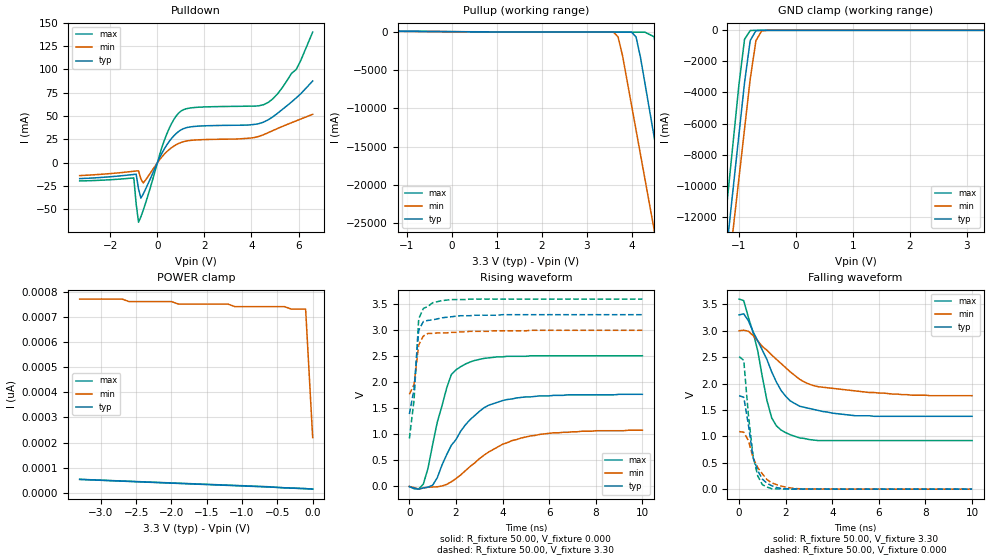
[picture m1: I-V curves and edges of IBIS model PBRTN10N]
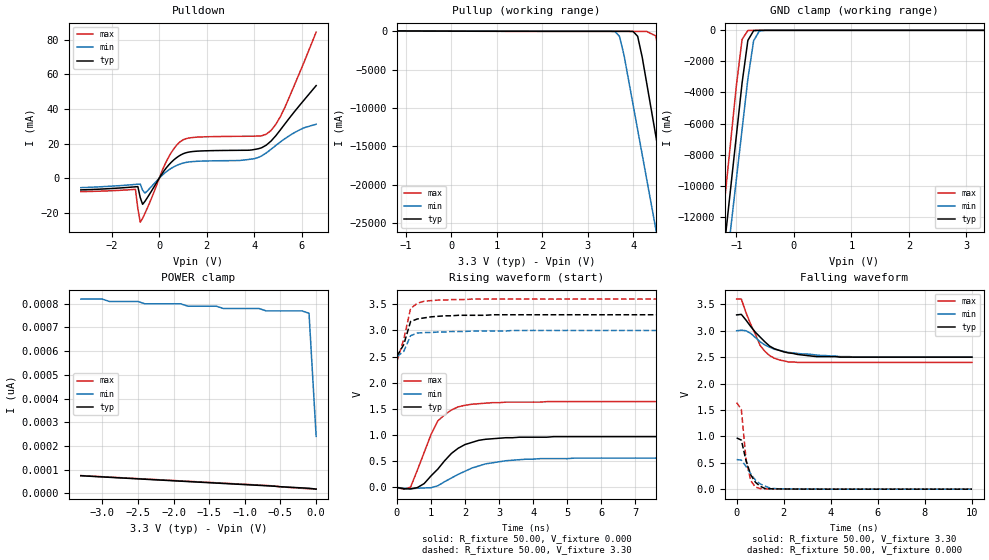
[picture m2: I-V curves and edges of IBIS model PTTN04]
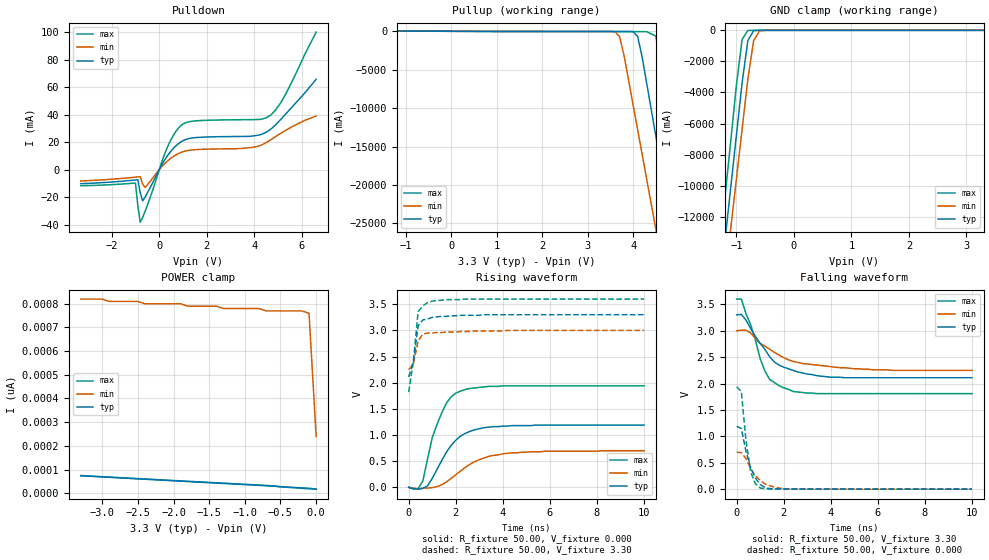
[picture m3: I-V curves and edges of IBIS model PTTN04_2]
| Integrated Devices Technolgy, Inc.
| IBIS MODEL OF 82v2048E
| BGA_208
[Ibis Ver]   2.1
[File Name]   2048E_02.ibs
[File Rev]   1.0
[Date]   10/24/2002
[Source]   Integrated Devices Technolgy, Inc.
[Notes]   Spice type : spectre
[Disclaimer] Integrated Device Technology, Inc. ("IDT") hereby grants the
   user of this IBIS model a non-exclusive, nontransferable
   license to use this IBIS model under the following terms. The
   user is granted this license only to use the IBIS model and is
   not granted rights to sell, copy (except as needed to run the
   IBIS model), rent, lease or sub-license the IBIS model in
   whole or in part, or in modified form to anyone. The User may
   modify the IBIS model to suit its specific applications, but
   rights to derivative works and such modifications shall belong
   to IDT. This IBIS model is provided on an AS IS" basis and IDT
   makes absolutely no warranty with respect to the information
   contained herein. IDT DISCLAIMS AND CUSTOMER WAIVES ALL
   WARRANTIES, EXPRESS AND IMPLIED, INCLUDING WARRANTIES OF
   MERCHANTABILITY AND FITNESS FOR A PARTICULAR PURPOSE. THE
   ENTIRE RISK AS TO QUALITY AND PERFORMANCE IS WITH THE USER
   ACCORDINGLY, IN NO EVENT SHALL IDT BE LIABLE FOR ANY DIRECT OR
   INDIRECT DAMAGES, WHETHER IN CONTRACT OR TORT, INCLUDING ANY
   LOST PROFITS OR OTHER INCIDENTAL, CONSEQUENTIAL, EXEMPLARY, OR
   PUNITIVE DAMAGES ARISING OUT OF THE USE OR APPLICATION OF THE
   IBIS model. Further, IDT reserves the right to make changes
   without notice to any product herein to improve reliability,
   function, or design. IDT does not convey any license under
   patent rights or any other intellectual property rights,
   including those of third parties. IDT is not obligated to
   provide maintenance or support for the licensed IBIS model.
[Copyright]   Copyright 2002, Integrated Devices Technolgy, Inc. all rights
   reserved
|   Component 2048E_02 (BGA_208)
[Component]   2048E_02
[Manufacturer]   Integrated Devices Technolgy, Inc.
[Package]
| variable   typ   min   max
R_pkg   169.8m   150.2m   189.4m
L_pkg   4.44nH   3.68nH   5.19nH
C_pkg   0.81pF   0.54pF   1.08pF
|   Pin List ( BGA_208 )
[PIN]   signal_name   Model_name   R_pin   L_pin   C_pin
   A1   GNDA   GND
   A2   GNDT4   GND
   A3   TTIP4   DRIVER
   A4   VDDT   POWER
   A5   RTIP4   PAI
   A6   TRST   PITSU
   A7   GNDT2   GND
   A8   TTIP2   DRIVER
   A9   VDDT   POWER
   A10   TCK   PITSN
   A11   RTIP2   PAI
   A12   GNDT1   GND
   A13   TTIP1   DRIVER
   A14   VDDT   POWER
   A15   TCLK1   PITSN
   A16   RCLK1   PTTN04_2
   B1   SCLKE   PITSN
   B2   GNDT12   GND
   B3   TRING4   DRIVER
   B4   VDDT   POWER
   B5   RRING4   PAI
   B6   TMS   PITSU
   B7   GNDT10   GND
   B8   TRING2   DRIVER
   B9   VDDT   POWER
   B10   TDO   PTTN04
   B11   RRING2   PAI
   B12   GNDT9   GND
   B13   TRING1   DRIVER
   B14   VDDT   POWER
   B15   TD1/TDP1   PITSN
   B16   RD1/RDP1   PTTN04
   C1   VDDA   POWER
   C2   LOS1   POTN04
   C3   LOS2   POTN04
   C4   VDDR4   POWER
   C5   RTIP3   PAI
   C6   GNDR4   GND
   C7   GNDT3   GND
   C8   TTIP3   DRIVER
   C9   VDDT   POWER
   C10   VDDR2   POWER
   C11   RTIP1   PAI
   C12   GNDR2   GND
   C13   NC   NC
   C14   TDN1   PITSN
   C15   CV1/RDN1   PTTN04
   C16   TCLK2   PITSN
   D1   LOS3   POTN04
   D2   LOS4   POTN04
   D3   LOS5   POTN04
   D4   VDDR3   POWER
   D5   RRING3   PAI
   D6   GNDR3   GND
   D7   GNDT11   GND
   D8   TRING3   DRIVER
   D9   VDDT   POWER
   D10   VDDR1   POWER
   D11   RRING1   PAI
   D12   GNDR1   GND
   D13   TDI   PITSU
   D14   TDN2   PITSN
   D15   TD2/TDP2   PITSN
   D16   RCLK2   PTTN04_2
   E1   LOS6   POTN04
   E2   LOS7   POTN04
   E3   LOS8   POTN04
   E4   THZ   PITSN
   E13   CV2/RDN2   PTTN04
   E14   RD2/RDP2   PTTN04
   E15   TD3/TDP3   PITSN
   E16   TCLK3   PITSN
   F1   VDDD   POWER
   F2   INT/MOT   PITSN
   F3   IC   PITSN
   F4   GNDD   GND
   F13   TDN3   PITSN
   F14   CV3/RDN3   PTTN04
   F15   RD3/RDP3   PTTN04
   F16   RCLK3   PTTN04_2
   G1   MCLK   PITSN
   G2   GPIO0   PBRTN10N
   G3   GPIO1   PBRTN10N
   G4   P/S   PITSN
   G7   GNDA   GND
   G8   NC   NC
   G9   VDDIO   POWER
   G10   VDDIO   POWER
   G13   GNDD   GND
   G14   TDN4   PITSN
   G15   TD4/TDP4   PITSN
   G16   TCLK4   PITSN
   H1   VDDIO   POWER
   H2   D6   PBRTN10N
   H3   D7   PBRTN10N
   H4   GNDIO   GND
   H7   GNDA   GND
   H8   GNDA   GND
   H9   NC   NC
   H10   NC   NC
   H13   CV4/RDN4   PTTN04
   H14   RD4/RDP4   PTTN04
   H15   RCLK4   PTTN04_2
   H16   VDDD   POWER
   J1   D5   PBRTN10N
   J2   D4   PBRTN10N
   J3   D3   PBRTN10N
   J4   D2   PBRTN10N
   J7   GNDA   GND
   J8   GNDA   GND
   J9   GNDIO   GND
   J10   GNDIO   GND
   J13   GNDIO   GND
   J14   TDN5   PITSN
   J15   TD5/TDP5   PITSN
   J16   TCLK5   PITSN
   K1   VDDIO   POWER
   K2   D0   PBRTN10N
   K3   D1   PBRTN10N
   K4   GNDIO   GND
   K7   GNDA   GND
   K8   GNDA   GND
   K9   GNDA   GND
   K10   GNDA   GND
   K13   CV5/RDN5   PTTN04
   K14   RD5/RDP5   PTTN04
   K15   RCLK5   PTTN04_2
   K20   VDDIO   POWER
   L1   A7   PITSN
   L2   A6   PITSN
   L3   A5   PITSN
   L4   A4   PITSN
   L13   TESTV   PAO
   L14   TDN6   PITSN
   L15   TD6/TDP6   PITSN
   L16   TCLK6   PITSN
   M1   A0   PITSN
   M2   A1   PITSN
   M3   A2   PITSN
   M4   A3   PITSN
   M13   TDN7   PITSN
   M14   CV6/RDN6   PTTN04
   M15   RD6/RDP6   PTTN04
   M16   RCLK6   PTTN04_2
   N1   CS   PITSN
   N2   SCLK   PITSN
   N3   DS/RD   PITSN
   N4   VDDR6   POWER
   N5   RRING6   PAI
   N6   GNDR6   GND
   N7   GNDT6   GND
   N8   TRING6   DRIVER
   N9   VDDT   POWER
   N10   VDDR8   POWER
   N11   RRING8   PAI
   N12   GNDR8   GND
   N13   CV7/RDN7   PTTN04
   N14   RD7/RDP7   PTTN04
   N15   TD7/TDP7   PITSN
   N16   TCLK7   PITSN
   P1   SDI/RW/WR   PITSN
   P2   SDO   PTTN04_2
   P3   RST   PITSU
   P4   VDDR5   POWER
   P5   RTIP6   PAI
   P6   GNDR5   GND
   P7   GNDT14   GND
   P8   TTIP6   DRIVER
   P9   VDDT   POWER
   P10   VDDR7   POWER
   P11   RTIP8   PAI
   P12   GNDR7   GND
   P13   TESTSE   PITSN
   P14   RD8/RDP8   PTTN04
   P15   TDN8   PITSN
   P16   RCLK7   PTTN04_2
   R1   INT   POTN04
   R2   GNDT5   GND
   R3   TRING5   DRIVER
   R4   VDDT   POWER
   R5   RRING5   PAI
   R6   MCLKS   PITSN
   R7   GNDT7   GND
   R8   TRING7   DRIVER
   R9   VDDT   POWER
   R10   TESTAPLL   POTN04
   R11   RRING7   PAI
   R12   GNDT8   GND
   R13   TRING8   DRIVER
   R14   VDDT   POWER
   R15   CV8/RDN8   PTTN04
   R16   TD8/TDP8   PITSN
   T1   REF   PAO
   T2   GNDT13   GND
   T3   TTIP5   DRIVER
   T4   VDDT   POWER
   T5   RTIP5   PAI
   T6   GNDA   GND
   T7   GNDT15   GND
   T8   TTIP7   DRIVER
   T9   VDDT   POWER
   T10   VDDA   POWER
   T11   RTIP7   PAI
   T12   GNDT16   GND
   T13   TTIP8   DRIVER
   T14   VDDT   POWER
   T15   RCLK8   PTTN04_2
   T16   TCLK8   PITSN
| Models and submodels in the file (9): PBRTN10N (I/O), PTTN04 (3-state), PTTN04_2 (3-state), POTN04 (Output), PITSN (Input), PAI (Input), PITSU (Input), PAO (Input), DRIVER (3-state)
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|   Model PBRTN10N
[Model]   PBRTN10N
Model_type   I/O
Polarity   Non-Inverting
Enable   Active-Low
Vinl =   0.74V
Vinh =   2.10V
C_comp   3.50pF   4.00pF   3.20pF
[Temperature Range]   25.00   85.00   -40.00
[Voltage Range]   3.30V   3.00V   3.60V
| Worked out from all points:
|   slope of the pulldown table from 0 to 0.495 V, typ, clamps not added: 21.9 ohm
|   slope of the pullup table from 0 to 0.495 V, typ, clamps not added: 29.2 ohm
|   GND clamp passes 1 mA (typ) near -0.60 V on its own axis
|   rising waveform, R_fixture 50.00, V_fixture 0.000: 20-80 % time 1.59ns typ, 2.13ns min, 825ps max; typ from -0.002 V to 1.77 V
|   rising waveform, R_fixture 50.00, V_fixture 3.30: 20-80 % time 226ps typ, 225ps min, 235ps max; typ from 1.39 V to 3.3 V
|   falling waveform, R_fixture 50.00, V_fixture 3.30: 20-80 % time 1.32ns typ, 1.97ns min, 801ps max; typ from 3.3 V to 1.38 V
|   falling waveform, R_fixture 50.00, V_fixture 0.000: 20-80 % time 472ps typ, 702ps min, 384ps max; typ from 1.77 V to 0 V
[Pulldown]
| voltage   I(typ)   I(min)   I(max)
-3.3V     -16.95mA   -13.71mA   -19.45mA
-1V       -12.5mA    -9.06mA    -16.2mA
-900mV    -12.2mA    -8.75mA    -44.01mA
-800mV    -27.97mA   -8.57mA    -63.62mA
-700mV    -37.8mA    -17.39mA   -57.93mA
-600mV    -33.43mA   -21.55mA   -50.78mA
300mV     15.03mA    9.35mA     24.27mA
900mV     33.46mA    20.65mA    53.15mA
1.5V      38.77mA    24.19mA    59.03mA
4.7V      45.89mA    32.14mA    64.49mA
5.9V      69.46mA    44.93mA    100mA
6.6V      87.62mA    51.95mA    140mA
[Pullup]
| voltage   I(typ)   I(min)   I(max)
-3.3V     120mA      79.67mA    180mA
3.6V      -41.5mA    -64.51mA   -72.86mA
3.7V      -41.65mA   -690mA     -73.1mA
3.8V      -41.8mA    -3.15A     -73.33mA
4.1V      -690mA     -12.84A    -73.96mA
4.3V      -6.82A     -19.3A     -75.1mA
4.5V      -13.65A    -25.76A    -660mA
4.7V      -20.47A    -32.21A    -7.27A
4.9V      -27.29A    -38.67A    -14.54A
5.1V      -34.12A    -45.13A    -21.81A
5.3V      -40.94A    -51.59A    -29.07A
6.6V      -85.3A     -93.57A    -76.32A
[GND_clamp]
| voltage   I(typ)   I(min)   I(max)
-3.3V     -85.25A    -83.86A    -87.14A
-1.3V     -17.02A    -19.27A    -14.46A
-1.2V     -13.61A    -16.05A    -10.83A
-1.1V     -10.19A    -12.82A    -7.2A
-1V       -6.78A     -9.59A     -3.56A
-900mV    -3.37A     -6.36A     -580mA
-800mV    -650mA     -3.13A     -10.84mA
-700mV    -23.03mA   -670mA     -750uA
-600mV    -570uA     -40.72mA   -46.43uA
-400mV    -420nA     -76.92uA   -33.22nA
3.3V      15.23pA    730pA      12.85pA
[POWER_clamp]
| voltage   I(typ)   I(min)   I(max)
-3.3V     53.95pA    770pA      54.34pA
-2.7V     47.02pA    770pA      47.72pA
-2.6V     45.88pA    760pA      46.62pA
-2V       39.11pA    760pA      40.01pA
-1.9V     37.99pA    750pA      38.91pA
-1.2V     30.19pA    750pA      31.21pA
-1.1V     29.08pA    740pA      30.11pA
-400mV    20.85pA    740pA      20.54pA
-300mV    19.76pA    730pA      19.3pA
-100mV    17.59pA    730pA      17.04pA
0V        15.23pA    220pA      15.99pA
[Ramp]
| variable   typ   min   max
dV/dt_r   1.06/1.42n   0.65/2.13n   1.51/0.80n
dV/dt_f   1.15/1.32n   0.74/1.94n   1.61/0.81n
R_load = 50.00
[Rising Waveform]
R_fixture = 50.00
V_fixture = 0.000
V_fixture_min = 0.000
V_fixture_max = 0.000
| time   V(typ)   V(min)   V(max)
0s        -2.35mV    -1.01mV    -3.76mV
600ps     -28.68mV   -31.05mV   45.89mV
1ns       23.7mV     -11.09mV   810mV
1.6ns     610mV      39.29mV    1.89V
1.8ns     790mV      88.39mV    2.15V
2.2ns     1.06V      220mV      2.3V
3.2ns     1.51V      600mV      2.46V
4.2ns     1.67V      840mV      2.5V
6.2ns     1.75V      1.03V      2.51V
10ns      1.77V      1.08V      2.51V
[Rising Waveform]
R_fixture = 50.00
V_fixture = 3.30
V_fixture_min = 3.00
V_fixture_max = 3.60
| time   V(typ)   V(min)   V(max)
0s        1.39V      1.77V      920mV
200ps     1.87V      1.96V      1.66V
400ps     3V         2.72V      3.22V
600ps     3.17V      2.89V      3.42V
800ps     3.19V      2.94V      3.46V
1ns       3.2V       2.94V      3.53V
1.8ns     3.26V      2.96V      3.59V
2.8ns     3.29V      2.98V      3.6V
5.2ns     3.3V       3V         3.6V
10ns      3.3V       3V         3.6V
[Falling Waveform]
R_fixture = 50.00
V_fixture = 3.30
V_fixture_min = 3.00
V_fixture_max = 3.60
| time   V(typ)   V(min)   V(max)
0s        3.3V       3V         3.6V
200ps     3.32V      3.01V      3.57V
600ps     2.98V      2.91V      2.97V
800ps     2.81V      2.81V      2.62V
1.2ns     2.45V      2.63V      1.67V
1.4ns     2.22V      2.54V      1.35V
1.8ns     1.87V      2.38V      1.12V
2.6ns     1.57V      2.08V      970mV
3.4ns     1.49V      1.94V      920mV
10ns      1.38V      1.77V      920mV
[Falling Waveform]
R_fixture = 50.00
V_fixture = 0.000
V_fixture_min = 0.000
V_fixture_max = 0.000
| time   V(typ)   V(min)   V(max)
0s        1.77V      1.09V      2.51V
200ps     1.74V      1.08V      2.44V
400ps     1.22V      920mV      1.4V
600ps     600mV      590mV      630mV
800ps     350mV      410mV      250mV
1ns       190mV      290mV      86.54mV
1.4ns     65.04mV    120mV      8.44mV
1.8ns     15.51mV    59.38mV    3.46mV
2.4ns     4.08mV     13.27mV    1.63mV
10ns      1.37uV     -16.49uV   -7.85uV
|   Model PTTN04
[Model]   PTTN04
Model_type   3-state
Polarity   Non-Inverting
Enable   Active-Low
C_comp   3.50pF   4.00pF   3.50pF
[Temperature Range]   25.00   85.00   -40.00
[Voltage Range]   3.30V   3.00V   3.60V
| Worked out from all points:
|   slope of the pulldown table from 0 to 0.495 V, typ, clamps not added: 54.8 ohm
|   slope of the pullup table from 0 to 0.495 V, typ, clamps not added: 58.3 ohm
|   GND clamp passes 1 mA (typ) near -0.60 V on its own axis
|   rising waveform, R_fixture 50.00, V_fixture 0.000: 20-80 % time 911ps typ, 1.18ns min, 672ps max; typ from -0.001 V to 0.97 V
|   rising waveform, R_fixture 50.00, V_fixture 3.30: 20-80 % time 244ps typ, 200ps min, 267ps max; typ from 2.51 V to 3.3 V
|   falling waveform, R_fixture 50.00, V_fixture 3.30: 20-80 % time 1.1ns typ, 1.37ns min, 761ps max; typ from 3.3 V to 2.5 V
|   falling waveform, R_fixture 50.00, V_fixture 0.000: 20-80 % time 430ps typ, 596ps min, 274ps max; typ from 0.97 V to 0 V
[Pulldown]
| voltage   I(typ)   I(min)   I(max)
-3.3V     -6.78mA    -5.48mA    -7.78mA
-1V       -5mA       -3.62mA    -6.48mA
-900mV    -4.88mA    -3.5mA     -17.6mA
-800mV    -11.19mA   -3.43mA    -25.45mA
-700mV    -15.12mA   -6.95mA    -23.17mA
-600mV    -13.37mA   -8.62mA    -20.31mA
300mV     6.01mA     3.74mA     9.71mA
900mV     13.39mA    8.26mA     21.26mA
3.9V      16.33mA    11.07mA    24.26mA
4.7V      21.41mA    16.66mA    27.53mA
5.3V      31.61mA    22.97mA    41.38mA
6.6V      53.5mA     31.16mA    84.43mA
[Pullup]
| voltage   I(typ)   I(min)   I(max)
-3.3V     75.1mA     45.9mA     110mA
3.6V      -20.75mA   -52.61mA   -36.43mA
3.7V      -20.82mA   -680mA     -36.55mA
3.8V      -20.91mA   -3.14A     -36.66mA
4.1V      -670mA     -12.83A    -36.98mA
4.3V      -6.8A      -19.29A    -37.92mA
4.5V      -13.63A    -25.74A    -620mA
4.7V      -20.45A    -32.2A     -7.23A
4.9V      -27.27A    -38.66A    -14.5A
5.1V      -34.1A     -45.12A    -21.77A
5.3V      -40.92A    -51.58A    -29.04A
6.6V      -85.27A    -93.56A    -76.28A
[GND_clamp]
| voltage   I(typ)   I(min)   I(max)
-3.3V     -85.25A    -83.86A    -87.14A
-1.3V     -17.02A    -19.27A    -14.46A
-1.2V     -13.61A    -16.05A    -10.83A
-1.1V     -10.19A    -12.82A    -7.2A
-1V       -6.78A     -9.59A     -3.56A
-900mV    -3.37A     -6.36A     -580mA
-800mV    -650mA     -3.13A     -10.84mA
-700mV    -23.03mA   -670mA     -750uA
-600mV    -570uA     -40.72mA   -46.43uA
-400mV    -420nA     -76.92uA   -33.22nA
3.3V      17.37pA    770pA      12.87pA
[POWER_clamp]
| voltage   I(typ)   I(min)   I(max)
-3.3V     73.8pA     820pA      74.49pA
-2.5V     60.59pA    810pA      61.66pA
-2.4V     58.95pA    800pA      60.06pA
-1.9V     50.83pA    800pA      52.05pA
-1.8V     49.21pA    790pA      50.45pA
-1.4V     42.75pA    790pA      44.05pA
-1.3V     41.14pA    780pA      42.44pA
-800mV    33.09pA    780pA      34.44pA
-700mV    31.48pA    770pA      32.83pA
-200mV    22.54pA    770pA      20.69pA
-100mV    20.96pA    760pA      18.49pA
0V        17.27pA    240pA      17.07pA
[Ramp]
| variable   typ   min   max
dV/dt_r   0.58/0.86n   0.34/1.22n   0.98/0.61n
dV/dt_f   0.48/1.02n   0.30/1.52n   0.72/0.71n
R_load = 50.00
[Rising Waveform]
R_fixture = 50.00
V_fixture = 0.000
V_fixture_min = 0.000
V_fixture_max = 0.000
| time   V(typ)   V(min)   V(max)
0s        -1.28mV    -400uV     -2.34mV
200ps     -25mV      -16.44mV   -33.49mV
400ps     -28.55mV   -25.32mV   4.49mV
800ps     73.89mV    -10.55mV   670mV
1ns       220mV      -5.62mV    1.01V
1.2ns     350mV      31.07mV    1.27V
1.8ns     750mV      250mV      1.54V
2.4ns     900mV      410mV      1.6V
3.8ns     960mV      540mV      1.63V
10ns      970mV      560mV      1.64V
[Rising Waveform]
R_fixture = 50.00
V_fixture = 3.30
V_fixture_min = 3.00
V_fixture_max = 3.60
| time   V(typ)   V(min)   V(max)
0s        2.51V      2.5V       2.41V
200ps     2.73V      2.6V       2.83V
400ps     3.17V      2.9V       3.42V
600ps     3.22V      2.95V      3.52V
800ps     3.24V      2.96V      3.56V
1.4ns     3.28V      2.97V      3.58V
2.2ns     3.29V      2.99V      3.6V
2.8ns     3.3V       2.99V      3.6V
3.4ns     3.3V       3V         3.6V
10ns      3.3V       3V         3.6V
[Falling Waveform]
R_fixture = 50.00
V_fixture = 3.30
V_fixture_min = 3.00
V_fixture_max = 3.60
| time   V(typ)   V(min)   V(max)
0s        3.3V       3V         3.6V
200ps     3.31V      3.01V      3.6V
600ps     3.08V      2.95V      3.12V
1ns       2.88V      2.79V      2.72V
1.4ns     2.71V      2.69V      2.53V
1.8ns     2.63V      2.63V      2.45V
2.2ns     2.58V      2.59V      2.41V
3.4ns     2.51V      2.54V      2.4V
5ns       2.5V       2.5V       2.4V
10ns      2.5V       2.5V       2.4V
[Falling Waveform]
R_fixture = 50.00
V_fixture = 0.000
V_fixture_min = 0.000
V_fixture_max = 0.000
| time   V(typ)   V(min)   V(max)
0s        970mV      560mV      1.64V
200ps     930mV      550mV      1.51V
400ps     540mV      430mV      560mV
600ps     270mV      290mV      160mV
800ps     130mV      170mV      38.48mV
1ns       56mV       100mV      11.04mV
1.2ns     12.7mV     59.65mV    7.28mV
1.4ns     7.26mV     23.89mV    4.27mV
1.8ns     4.54mV     6.11mV     1.29mV
10ns      1.93uV     9.71uV     820nV
|   Model PTTN04_2
[Model]   PTTN04_2
Model_type   3-state
Polarity   Non-Inverting
Enable   Active-Low
C_comp   3.50pF   4.00pF   3.50pF
[Temperature Range]   25.00   85.00   -40.00
[Voltage Range]   3.30V   3.00V   3.60V
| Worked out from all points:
|   slope of the pulldown table from 0 to 0.495 V, typ, clamps not added: 36.6 ohm
|   slope of the pullup table from 0 to 0.495 V, typ, clamps not added: 46.6 ohm
|   GND clamp passes 1 mA (typ) near -0.60 V on its own axis
|   rising waveform, R_fixture 50.00, V_fixture 0.000: 20-80 % time 1.05ns typ, 1.49ns min, 812ps max; typ from -0.002 V to 1.19 V
|   rising waveform, R_fixture 50.00, V_fixture 3.30: 20-80 % time 233ps typ, 259ps min, 255ps max; typ from 2.11 V to 3.3 V
|   falling waveform, R_fixture 50.00, V_fixture 3.30: 20-80 % time 1.24ns typ, 1.8ns min, 816ps max; typ from 3.3 V to 2.11 V
|   falling waveform, R_fixture 50.00, V_fixture 0.000: 20-80 % time 481ps typ, 664ps min, 314ps max; typ from 1.19 V to 0 V
[Pulldown]
| voltage   I(typ)   I(min)   I(max)
-3.3V     -10.17mA   -8.22mA    -11.67mA
-1V       -7.5mA     -5.43mA    -9.72mA
-900mV    -7.32mA    -5.25mA    -26.41mA
-800mV    -16.78mA   -5.14mA    -38.17mA
-700mV    -22.68mA   -10.43mA   -34.76mA
-600mV    -20.06mA   -12.93mA   -30.47mA
300mV     9.02mA     5.61mA     14.56mA
800mV     18.81mA    11.62mA    30.08mA
1.3V      22.8mA     14.17mA    34.98mA
4.7V      29.57mA    21.83mA    39.85mA
5.3V      40.09mA    28.41mA    54.3mA
6.6V      65.68mA    39.04mA    100mA
[Pullup]
| voltage   I(typ)   I(min)   I(max)
-3.3V     86.33mA    53.19mA    130mA
3.6V      -25.94mA   -55.59mA   -45.54mA
3.7V      -26.03mA   -680mA     -45.69mA
3.8V      -26.13mA   -3.14A     -45.83mA
4.1V      -680mA     -12.83A    -46.23mA
4.3V      -6.81A     -19.29A    -47.22mA
4.5V      -13.63A    -25.75A    -630mA
4.7V      -20.46A    -32.21A    -7.24A
4.9V      -27.28A    -38.66A    -14.51A
5.1V      -34.1A     -45.12A    -21.78A
5.3V      -40.93A    -51.58A    -29.05A
6.6V      -85.28A    -93.56A    -76.29A
[GND_clamp]
| voltage   I(typ)   I(min)   I(max)
-3.3V     -85.25A    -83.86A    -87.14A
-1.3V     -17.02A    -19.27A    -14.46A
-1.2V     -13.61A    -16.05A    -10.83A
-1.1V     -10.19A    -12.82A    -7.2A
-1V       -6.78A     -9.59A     -3.56A
-900mV    -3.37A     -6.36A     -580mA
-800mV    -650mA     -3.13A     -10.84mA
-700mV    -23.03mA   -670mA     -750uA
-600mV    -570uA     -40.72mA   -46.43uA
-400mV    -420nA     -76.92uA   -33.22nA
3.3V      17.37pA    770pA      12.85pA
[POWER_clamp]
| voltage   I(typ)   I(min)   I(max)
-3.3V     73.8pA     820pA      74.44pA
-2.5V     60.58pA    810pA      61.62pA
-2.4V     58.95pA    800pA      60.02pA
-1.9V     50.82pA    800pA      52.01pA
-1.8V     49.21pA    790pA      50.41pA
-1.4V     42.75pA    790pA      44.01pA
-1.3V     41.13pA    780pA      42.41pA
-800mV    33.09pA    780pA      34.41pA
-700mV    31.48pA    770pA      32.8pA
-200mV    22.54pA    770pA      20.66pA
-100mV    20.96pA    760pA      18.46pA
0V        17.27pA    240pA      17.04pA
[Ramp]
| variable   typ   min   max
dV/dt_r   0.72/1.04n   0.42/1.49n   1.17/0.70n
dV/dt_f   0.71/1.19n   0.45/1.73n   1.07/0.81n
R_load = 50.00
[Rising Waveform]
R_fixture = 50.00
V_fixture = 0.000
V_fixture_min = 0.000
V_fixture_max = 0.000
| time   V(typ)   V(min)   V(max)
0s        -1.51mV    -530uV     -2.62mV
400ps     -35.79mV   -32.19mV   -25.03mV
600ps     -19.18mV   -19.59mV   120mV
1ns       170mV      -7.41mV    950mV
1.4ns     510mV      48.34mV    1.42V
1.8ns     800mV      170mV      1.73V
2.2ns     980mV      310mV      1.84V
3ns       1.12V      530mV      1.91V
4ns       1.17V      640mV      1.94V
10ns      1.19V      700mV      1.94V
[Rising Waveform]
R_fixture = 50.00
V_fixture = 3.30
V_fixture_min = 3.00
V_fixture_max = 3.60
| time   V(typ)   V(min)   V(max)
0s        2.11V      2.25V      1.82V
200ps     2.41V      2.36V      2.41V
400ps     3.09V      2.8V       3.36V
600ps     3.2V       2.93V      3.47V
800ps     3.22V      2.95V      3.53V
1ns       3.25V      2.95V      3.56V
1.6ns     3.27V      2.97V      3.59V
2.2ns     3.29V      2.98V      3.59V
3.2ns     3.3V       2.99V      3.6V
10ns      3.3V       3V         3.6V
[Falling Waveform]
R_fixture = 50.00
V_fixture = 3.30
V_fixture_min = 3.00
V_fixture_max = 3.60
| time   V(typ)   V(min)   V(max)
0s        3.3V       3V         3.6V
200ps     3.31V      3.01V      3.6V
600ps     3.04V      2.96V      3.11V
1ns       2.76V      2.76V      2.47V
1.2ns     2.65V      2.71V      2.24V
1.4ns     2.51V      2.65V      2.08V
2ns       2.31V      2.49V      1.92V
2.4ns     2.25V      2.42V      1.85V
4ns       2.12V      2.32V      1.81V
10ns      2.11V      2.25V      1.81V
[Falling Waveform]
R_fixture = 50.00
V_fixture = 0.000
V_fixture_min = 0.000
V_fixture_max = 0.000
| time   V(typ)   V(min)   V(max)
0s        1.19V      700mV      1.94V
200ps     1.15V      690mV      1.85V
400ps     710mV      580mV      910mV
600ps     400mV      390mV      320mV
800ps     210mV      250mV      99.86mV
1ns       88.8mV     170mV      21.99mV
1.2ns     33.22mV    99.38mV    7.33mV
1.4ns     12.02mV    66.22mV    5.32mV
2.2ns     3.35mV     5.86mV     780uV
10ns      -1.47uV    2.87uV     780nV
